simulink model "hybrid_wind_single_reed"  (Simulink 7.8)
settings: Solver=FixedStepDiscrete  SolverMode=SingleTasking  StartTime=0.0  StopTime=inf  FixedStep=Ts  RelTol=1e-3
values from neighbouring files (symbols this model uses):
  amp_gain_factor = 0.73316    [hybrid_wind.m]    (also in measurements.m = 0.73312)
  gamma_cte = 0.7    [single_reed.m]
  HLL_d = c2d(HLL_c,Ts)    [hybrid_wind.m]    (also in measurements.m)
  maxoutputvoltage = 5    [hybrid_wind.m]    (also in measurements.m)
  micoffset_V = mean(voltsin_calib)    [hybrid_wind.m]    (also in measurements.m)
  micpreampsensitivity = -0.0025726    [hybrid_wind.m]    (also in measurements.m)
  PM = 50    [bowed_string_hyperbolic.m]    (also in lip_reed.m = 20; single_reed.m = 100)
  Ts = 25e-6    (= 2.5e-05)    [hybrid_wind.m]    (also in measurements.m)
  Zc = rho*c/St    (= 2615281.00417)    [hybrid_wind.m]
  zeta = 0.35    [single_reed.m]
undefined symbols (not defined in the file or in its folder): Bl, cell2mat, HRreed_G, HRreed_G_zm1, Mms, Re, Sd, sigbuilder_block
libraries: simulink x2

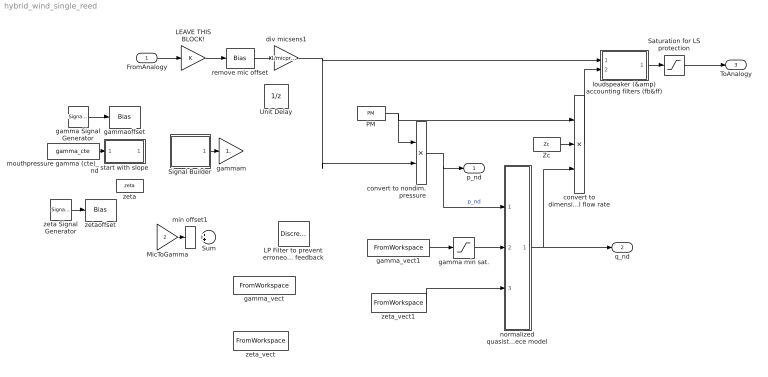
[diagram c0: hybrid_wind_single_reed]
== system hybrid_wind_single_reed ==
  FromAnalogy : Inport  Interpolate=off
  LEAVE THIS BLOCK! : Gain
  LP Filter to prevent erroneous high freq feedback : DiscreteFilter  Numerator=HdLP.ScaleValues(1)*HdLP.sosMatrix(1:end/2)  Denominator=HdLP.ScaleValues(2)*HdLP.sosMatrix(1+end/2:end)  SampleTime=Ts
  MicToGamma : Gain  Gain=2
  PM : Constant  Value=PM
  Saturation for LS protection : Saturate  UpperLimit=maxoutputvoltage  LowerLimit=-maxoutputvoltage
  Signal Builder : Subsystem  Tag=STV Subsys  LoadFcn=sigbuilder_block('load');  StartFcn=sigbuilder_block('start');  StopFcn=sigbuilder_block('stop');  ClipboardFcn=sigbuilder_block('clipboard');
  Sum : Sum  Inputs=++|
  Unit Delay : UnitDelay  SampleTime=-1
  Zc : Constant  Value=Zc
  convert to dimensional flow rate : Product  Inputs=*/*
  convert to nondim. pressure : Product  Inputs=/*
  div micsens1 : Gain  Gain=1/micpreampsensitivity
  gamma Signal Generator : SignalGenerator  WaveForm=sawtooth  Amplitude=(0.9-0.4)/2  Frequency=12
  gamma min sat. : Saturate  UpperLimit=100  LowerLimit=0.3333
  gamma_vect : FromWorkspace  VariableName=gamma_vect  SampleTime=0
  gamma_vect1 : FromWorkspace  VariableName=gamma_envs_all  SampleTime=0
  gammam : Gain  Gain=1.
  gammaoffset : Bias  Bias=0.4+(0.9-0.4)/2
  loudspeaker (&amp) accounting filters (fb&ff) : Subsystem
  min offset1 : Bias  Bias=-0.2
  mouthpressure gamma (cte)_nd : Constant  Value=gamma_cte
  normalized quasistatic mouthpiece model : Subsystem
  remove mic offset : Bias  Bias=-micoffset_V
  start with slope : Subsystem
  zeta : Constant  Value=zeta
  zeta Signal Generator : SignalGenerator  WaveForm=sawtooth  Amplitude=(0.3-0.1)/2  Frequency=10
  zeta_vect : FromWorkspace  VariableName=zeta_vect  SampleTime=0  OutputAfterFinalValue=Setting to zero
  zeta_vect1 : FromWorkspace  VariableName=zeta_envs_all_b  SampleTime=0  OutputAfterFinalValue=Setting to zero
  zetaoffset : Bias  Bias=0.1+(0.3-0.1)/2
  p_nd : Outport
  q_nd : Outport  Port=2
  ToAnalogy : Outport  Port=3
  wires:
  normalized quasistatic mouthpiece model/1(q_nd) -> q_nd/1, convert to dimensional flow rate/3
  convert to dimensional flow rate/1 -> loudspeaker (&amp) accounting filters (fb&ff)/2(q_calc)
  Zc/1 -> convert to dimensional flow rate/2
  convert to nondim. pressure/1 -> p_nd/1, normalized quasistatic mouthpiece model/1(p)  "p_nd"
  zeta Signal Generator/1 -> zetaoffset/1
  gamma Signal Generator/1 -> gammaoffset/1
  mouthpressure gamma (cte)_nd/1 -> start with slope/1(gamma_in)
  Signal Builder/1(Signal 1) -> gammam/1
  LEAVE THIS BLOCK!/1 -> remove mic offset/1
  loudspeaker (&amp) accounting filters (fb&ff)/1(V_amp_in) -> Saturation for LS protection/1
  FromAnalogy/1 -> LEAVE THIS BLOCK!/1
  MicToGamma/1 -> min offset1/1
  PM/1 -> convert to nondim. pressure/1, convert to dimensional flow rate/1
  gamma min sat./1 -> normalized quasistatic mouthpiece model/2(gamma)
  remove mic offset/1 -> div micsens1/1
  div micsens1/1 -> loudspeaker (&amp) accounting filters (fb&ff)/1(p), convert to nondim. pressure/2
  Saturation for LS protection/1 -> ToAnalogy/1
  gamma_vect1/1 -> gamma min sat./1
  zeta_vect1/1 -> normalized quasistatic mouthpiece model/3(zeta)

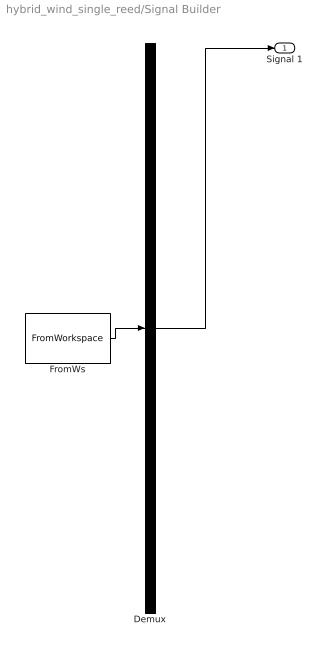
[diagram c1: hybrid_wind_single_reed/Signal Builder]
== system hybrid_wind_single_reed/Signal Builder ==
  Demux : Demux  Tag=STV Demux  Outputs=1
  FromWs : FromWorkspace  Tag=STV FromWs  VariableName=tuvar  SampleTime=0  SigBuilderData=DataTag0  VnvData=DataTag1
  Signal 1 : Outport  Tag=STV Outport
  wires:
  Demux/1 -> Signal 1/1
  FromWs/1 -> Demux/1

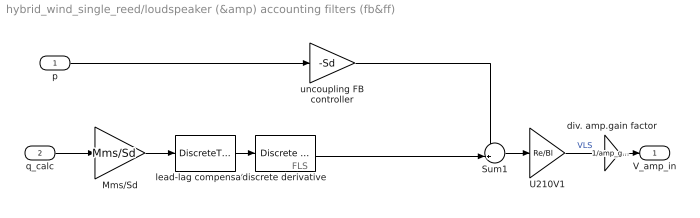
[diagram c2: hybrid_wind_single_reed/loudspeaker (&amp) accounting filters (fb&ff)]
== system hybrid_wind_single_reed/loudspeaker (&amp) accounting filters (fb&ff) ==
  note: FLS
  p : Inport
  q_calc : Inport  Port=2
  Mms/Sd : Gain  Gain=Mms/Sd
  Sum1 : Sum  Inputs=-+|
  U210V1 : Gain  Gain=Re/Bl
  discrete derivative : simulink/Discrete/Discrete Derivative  gainval=1.0  ICPrevScaledInput=0.0  InputProcessing=Inherited  OutMin=[]  OutMax=[]  OutDataType=fixdt(1, 16)  OutScaling=2^-10  DoSatur=off
  div. amp.gain factor : Gain  Gain=1/amp_gain_factor
  lead-lag compensator : DiscreteTransferFcn  Numerator=cell2mat(HLL_d.num)  Denominator=cell2mat(HLL_d.den)  SampleTime=Ts
  uncoupling FB controller : Gain  Gain=-Sd
  V_amp_in : Outport
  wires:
  q_calc/1 -> Mms/Sd/1
  uncoupling FB controller/1 -> Sum1/1
  div. amp.gain factor/1 -> V_amp_in/1
  p/1 -> uncoupling FB controller/1
  Mms/Sd/1 -> lead-lag compensator/1
  lead-lag compensator/1 -> discrete derivative/1
  Sum1/1 -> U210V1/1
  U210V1/1 -> div. amp.gain factor/1  "VLS"
  discrete derivative/1 -> Sum1/2

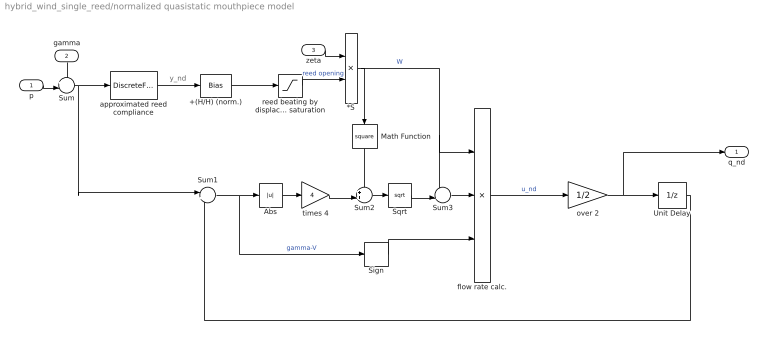
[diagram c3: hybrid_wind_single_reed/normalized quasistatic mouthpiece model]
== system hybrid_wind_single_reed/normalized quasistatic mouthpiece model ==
  note: y_nd
  p : Inport
  gamma : Inport  Port=2
  zeta : Inport  Port=3
  *S : Product  Inputs=**
  +(H/H) (norm.) : Bias  Bias=1
  Abs : Abs
  Math Function : Math  Operator=square
  Sign : Signum
  Sqrt : Sqrt
  Sum : Sum  Inputs=+-|  SampleTime=Ts
  Sum1 : Sum  Inputs=|++
  Sum2 : Sum  Inputs=++|
  Sum3 : Sum  Inputs=-+|
  Unit Delay : UnitDelay  SampleTime=-1
  approximated reed compliance : DiscreteFilter  Numerator=HRreed_G_zm1.num  Denominator=HRreed_G.den  SampleTime=Ts  a0EqualsOne=on
  flow rate calc. : Product  Inputs=3
  over 2 : Gain  Gain=1/2
  reed beating by displacement saturation : Saturate  UpperLimit=100  LowerLimit=0
  times 4 : Gain  Gain=4
  q_nd : Outport
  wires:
  gamma/1 -> Sum/1
  p/1 -> Sum/2
  zeta/1 -> *S/1
  Sum2/1 -> Sqrt/1
  Sum1/1 -> Abs/1, Sign/1  "gamma-V"
  Sum/1 -> Sum1/1, approximated reed compliance/1
  *S/1 -> flow rate calc./1, Sum3/1, Math Function/1  "W"
  flow rate calc./1 -> over 2/1  "u_nd"
  Sqrt/1 -> Sum3/2
  Sum3/1 -> flow rate calc./2
  over 2/1 -> q_nd/1, Unit Delay/1
  Math Function/1 -> Sum2/1
  Abs/1 -> times 4/1
  times 4/1 -> Sum2/2
  Sign/1 -> flow rate calc./3
  Unit Delay/1 -> Sum1/2
  approximated reed compliance/1 -> +(H/H) (norm.)/1
  +(H/H) (norm.)/1 -> reed beating by displacement saturation/1
  reed beating by displacement saturation/1 -> *S/2  "reed opening"

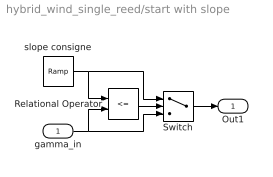
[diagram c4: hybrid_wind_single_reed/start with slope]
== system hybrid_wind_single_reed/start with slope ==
  gamma_in : Inport
  Relational Operator : RelationalOperator  Operator=<=  OutDataTypeStr=boolean
  Switch : Switch  Criteria=u2 > Threshold
  slope consigne : simulink/Sources/Ramp  slope=gamma_cte*1000  start=0  X0=0
  Out1 : Outport
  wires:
  slope consigne/1 -> Relational Operator/1, Switch/1
  gamma_in/1 -> Relational Operator/2, Switch/3
  Relational Operator/1 -> Switch/2
  Switch/1 -> Out1/1
